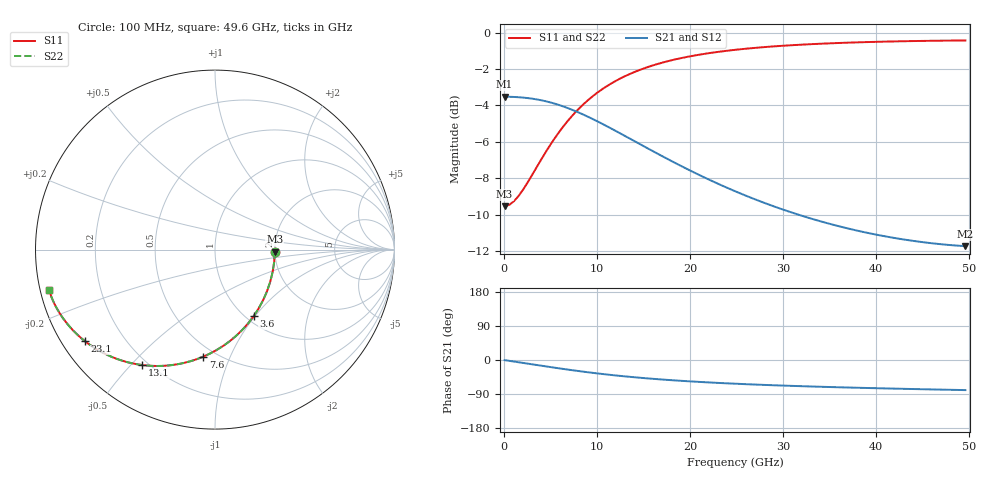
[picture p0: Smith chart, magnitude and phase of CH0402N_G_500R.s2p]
# GHz S RI R 500
! S-Parameters data
! Freq  reS11  imS11  reS21  imS21  reS12  imS12  reS22  imS22
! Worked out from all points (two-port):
!   100 points, 100 MHz to 49.6 GHz, reference 500 ohm
!   highest |S21| = -3.52 dB at 100 MHz (marker M1); lowest = -11.7 dB at 49.6 GHz (marker M2)
!   |S21| within 3 dB of the highest: start of sweep to 16.07 GHz
!   lowest |S11| = -9.5 dB at 100 MHz (marker M3), VSWR 2.00, Z = 999 - j25.6 ohm
!   |S11| at or under -10 dB: nowhere
!   |S22| runs from -9.5 to -0.4 dB; largest |S21 - S12| = 0
!   S11 on the Smith chart (normalised r, x): 100 MHz: 2.00, -0.05; 3.6 GHz: 1.08, -0.99; 7.6 GHz: 0.43, -0.80; 13.1 GHz: 0.18, -0.54; 23.1 GHz: 0.07, -0.32; 49.6 GHz: 0.03, -0.12
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0.1  0.3332 -0.0114  0.6666 -0.00431  0.6666 -0.00431  0.3332 -0.0114
0.6  0.3297 -0.0682  0.6659 -0.0258  0.6659 -0.0258  0.3297 -0.0682
1.6  0.3079 -0.1788  0.661 -0.0687  0.661 -0.0687  0.3079 -0.1788
2.6  0.2684 -0.2812  0.6515 -0.1108  0.6515 -0.1108  0.2684 -0.2812
3.6  0.2146 -0.372  0.6374 -0.1516  0.6374 -0.1516  0.2146 -0.372
4.6  0.1505 -0.449  0.6185 -0.1901  0.6185 -0.1901  0.1505 -0.449
5.6  0.0803 -0.5117  0.5956 -0.2254  0.5956 -0.2254  0.0803 -0.5117
6.6  0.00722 -0.5605  0.5692 -0.2566  0.5692 -0.2566  0.00722 -0.5605
7.6  -0.0658 -0.5967  0.5404 -0.2835  0.5404 -0.2835  -0.0658 -0.5967
8.6  -0.1368 -0.6219  0.5102 -0.3057  0.5102 -0.3057  -0.1368 -0.6219
10.6  -0.2677 -0.6462  0.449 -0.3372  0.449 -0.3372  -0.2677 -0.6462
13.1  -0.4059 -0.6431  0.3774 -0.3565  0.3774 -0.3565  -0.4059 -0.6431
14.6  -0.475 -0.6304  0.339 -0.3603  0.339 -0.3603  -0.475 -0.6304
16.6  -0.5531 -0.6065  0.2939 -0.3593  0.2939 -0.3593  -0.5531 -0.6065
19.6  -0.6448 -0.5636  0.2383 -0.3501  0.2383 -0.3501  -0.6448 -0.5636
23.1  -0.723 -0.5113  0.189 -0.3342  0.189 -0.3342  -0.723 -0.5113
25.1  -0.7573 -0.4824  0.1667 -0.3245  0.1667 -0.3245  -0.7573 -0.4824
28.6  -0.8045 -0.4351  0.1354 -0.308  0.1354 -0.308  -0.8045 -0.4351
33.1  -0.8479 -0.3806  0.1057 -0.2896  0.1057 -0.2896  -0.8479 -0.3806
37.1  -0.8755 -0.3377  0.0862 -0.2764  0.0862 -0.2764  -0.8755 -0.3377
41.6  -0.8981 -0.2945  0.0694 -0.2652  0.0694 -0.2652  -0.8981 -0.2945
49.6  -0.9239 -0.2268  0.0475 -0.2549  0.0475 -0.2549  -0.9239 -0.2268
